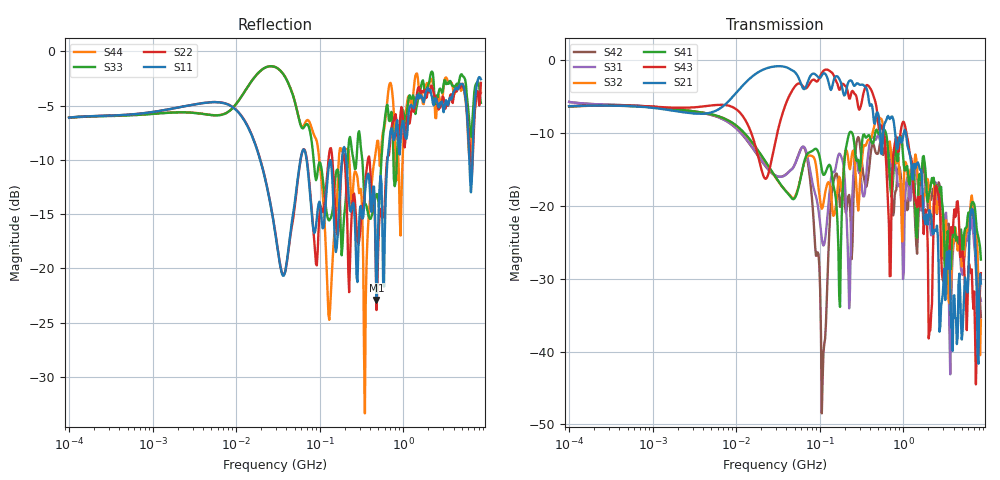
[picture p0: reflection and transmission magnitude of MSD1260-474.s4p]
# MHz S MA R 50
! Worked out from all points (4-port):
!   498 points, 100 kHz to 8.5 GHz, reference 50 ohm
!   strongest paths, dB at 100 kHz, 1.698 MHz, 29.49 MHz, 500.7 MHz, 8.5 GHz:
!     S21: -6.4, -6.9, -0.9, -7.4, -30.7
!     S43: -6.4, -6.5, -11.1, -8.6, -29.2
!     S41: -6.4, -6.7, -16.0, -10.0, -27.4
!     S32: -6.4, -6.7, -16.1, -7.8, -35.6
!     S31: -5.8, -6.7, -15.8, -10.3, -33.0
!     S42: -5.8, -6.7, -15.9, -12.8, -35.3
!   lowest |S11| = -22.9 dB at 478.3 MHz (marker M1), VSWR 1.15, Z = 55.6 - j5.06 ohm
!   |S11| at or under -10 dB: 69.7 MHz to 184.8 MHz (115.1 MHz wide, 90.5 % of centre); 207.5 MHz to 649.1 MHz (441.6 MHz wide, 103 % of centre); 6.183 GHz to 6.734 GHz (550.8 MHz wide, 8.53 % of centre)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
0.1  0.495 10.1  0.4811 10.0  0.5154 -10.6  0.4799 -171.0
     0.4811 10.0  0.495 10.3  0.4796 -171.1  0.5153 -10.8
     0.5154 -10.6  0.4796 -171.1  0.494 10.1  0.481 9.9
     0.4799 -171.0  0.5153 -10.8  0.481 9.9  0.4959 10.1
64.10508  0.3537 -8.8  0.6325 -15.8  0.2545 29.9  0.1928 -172.8
          0.6325 -15.8  0.3541 -8.0  0.1904 -171.1  0.2534 31.8
          0.2545 29.9  0.1904 -171.1  0.444 -45.6  0.6517 8.6
          0.1928 -172.8  0.2534 31.8  0.6517 8.6  0.4532 -46.1
110.9003  0.1537 -1.3  0.8083 -24.2  0.05335 148.7  0.1628 38.3
          0.8083 -24.2  0.183 7.2  0.1044 60.7  0.009896 78.3
          0.05335 148.7  0.1044 60.7  0.242 -57.4  0.8428 -8.2
          0.1628 38.3  0.009896 78.3  0.8428 -8.2  0.1975 -88.6
478.3074  0.07163 -39.2  0.4306 -89.5  0.2902 -24.1  0.3328 -34.7
          0.4306 -89.5  0.06434 -46.6  0.3949 -25.8  0.2276 -34.0
          0.2902 -24.1  0.3949 -25.8  0.2202 -22.2  0.4727 -121.1
          0.3328 -34.7  0.2276 -34.0  0.4727 -121.1  0.3669 -6.8
2159.325  0.6362 177.1  0.08697 91.0  0.06268 138.4  0.1446 144.0
          0.08697 91.0  0.6947 -177.4  0.07727 123.6  0.11 141.0
          0.06268 138.4  0.07727 123.6  0.8014 -175.1  0.01822 76.6
          0.1446 144.0  0.11 141.0  0.01822 76.6  0.7469 177.0
3568.796  0.6037 13.9  0.04919 148.6  0.01388 -119.1  0.05794 2.9
          0.04919 148.6  0.5981 14.1  0.02145 18.8  0.06067 -4.0
          0.01388 -119.1  0.02145 18.8  0.7276 11.5  0.04427 -68.1
          0.05794 2.9  0.06067 -4.0  0.04427 -68.1  0.7242 4.9
8500  0.7433 -54.7  0.02929 -103.4  0.0223 -100.1  0.04272 -130.4
      0.02929 -103.4  0.7156 -40.6  0.01652 -38.2  0.01715 -103.0
      0.0223 -100.1  0.01652 -38.2  0.5789 -47.2  0.03452 -58.7
      0.04272 -130.4  0.01715 -103.0  0.03452 -58.7  0.6438 -52.5
